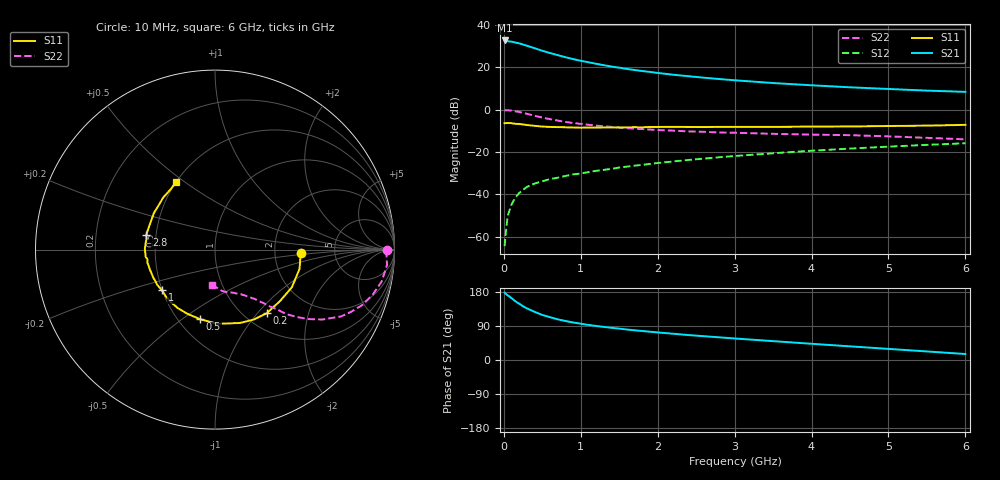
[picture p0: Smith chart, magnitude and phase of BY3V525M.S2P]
! SIEMENS Small Signal Semiconductors
! BFY420
! Si NPN RF SIEGET Grounded Emitter Transistor in MICRO-X
! VCE = 3.5 V  IC = 25 mA
! Common Emitter S-Parameters:  October  1996
# GHz  S  MA  R  50
!  f  S11  S21  S12  S22
! GHz  MAG  ANG  MAG  ANG  MAG  ANG  MAG  ANG
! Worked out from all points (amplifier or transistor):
!   36 points, 10 MHz to 6 GHz, reference 50 ohm
!   highest |S21| = 32.6 dB at 10 MHz (marker M1)
!   |S21| within 3 dB of that: start of sweep to 344.5 MHz
!   unconditionally stable (mu >= 1): start of sweep to 14.76 MHz; 1.772 GHz to end of sweep
!   at 250 MHz: K = 0.34, MSG = 34.3 dB, |S12| = -37.9 dB
!   at 1.4 GHz: K = 0.94, MSG = 24.1 dB, |S12| = -28.0 dB
!   at 6 GHz: K = 1.06, MAG = 10.7 dB, |S12| = -15.9 dB
!   S11 on the Smith chart (normalised r, x): 10 MHz: 2.82, -0.15; 200 MHz: 1.25, -1.12; 500 MHz: 0.64, -0.59; 1 GHz: 0.50, -0.26; 2.8 GHz: 0.44, +0.08; 6 GHz: 0.50, +0.47
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0.01  0.4773 -2.5  42.65 178.1  0.0006 98.5  0.9563 -0.2
0.02  0.4777 -5.1  42.25 175.2  0.001 84.6  0.9554 -1.4
0.1  0.4769 -26.2  39.87 163.3  0.0058 76.5  0.9452 -10.9
0.15  0.4617 -38.6  38.11 154.9  0.0084 74.8  0.9133 -16.0
0.2  0.4569 -51.0  36.34 148.5  0.0108 71.6  0.8785 -20.5
0.25  0.4454 -61.2  34.22 141.8  0.0127 67.8  0.8343 -24.5
0.3  0.4314 -71.4  32.05 136.2  0.015 67.3  0.7953 -27.9
0.4  0.4139 -88.1  28.02 127.1  0.018 63.2  0.7152 -33.0
0.5  0.3967 -101.9  24.37 118.9  0.0203 61.4  0.6477 -36.7
0.6  0.3894 -113.4  21.58 112.9  0.0229 61.1  0.5939 -39.3
0.7  0.3861 -122.7  19.23 107.4  0.0247 60.7  0.5498 -41.4
0.8  0.382 -130.3  17.17 102.9  0.0271 59.3  0.5122 -42.9
1  0.3726 -142.5  14.16 95.7  0.031 61.3  0.4593 -44.9
1.1  0.3768 -148.5  13.06 92.6  0.0336 61.1  0.4376 -46.2
1.4  0.3774 -160.0  10.31 84.9  0.0398 61.7  0.3904 -48.6
1.6  0.3808 -166.6  9.079 80.4  0.0451 60.6  0.3641 -50.4
2.2  0.3908 179.3  6.641 69.3  0.0597 59.4  0.3185 -55.2
2.8  0.3906 168.1  5.252 59.8  0.075 56.5  0.2877 -59.8
3.5  0.3901 156.6  4.224 49.8  0.0931 52.1  0.2677 -65.1
4.5  0.3995 141.5  3.349 36.0  0.12 44.2  0.2488 -73.6
5.5  0.4178 125.9  2.798 22.6  0.1471 35.3  0.2154 -86.1
6  0.4359 119.6  2.616 15.8  0.1603 30.5  0.1983 -94.1
